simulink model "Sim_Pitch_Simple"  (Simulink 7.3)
settings: Solver=ode23s  StartTime=0.0  StopTime=1000  RelTol=1e-3
InitFcn:
  | init
StartFcn:
  | init
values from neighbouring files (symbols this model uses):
  d2r = pi/180    (= 0.0174532925199)    [init.m]    (also in robust.m)
  r2d = 180/pi    (= 57.2957795131)    [init.m]    (also in robust.m)
undefined symbols (not defined in the file or in its folder): Aps, Bps, Cps, Dps, Kmix, Kq

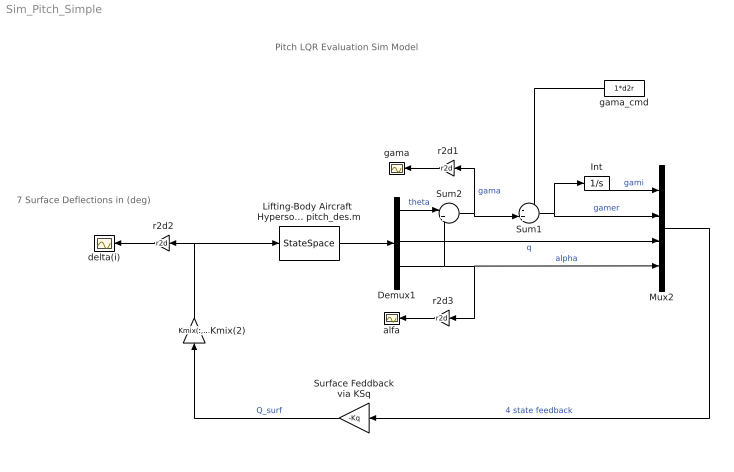
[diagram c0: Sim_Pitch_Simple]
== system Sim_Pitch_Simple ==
  note: 7 Surface Deflections in (deg)
  note: Pitch LQR Evaluation Sim Model
  " r2d1" : Gain  Gain=r2d  ParameterDataType=sfix(16)  ParameterScaling=2^0  OutDataType=sfix(16)  OutScaling=2^0
  " r2d2" : Gain  Gain=r2d  ParameterDataType=sfix(16)  ParameterScaling=2^0  OutDataType=sfix(16)  OutScaling=2^0
  " r2d3" : Gain  Gain=r2d  ParameterDataType=sfix(16)  ParameterScaling=2^0  OutDataType=sfix(16)  OutScaling=2^0
  Demux1 : Demux  Outputs=3
  Int : Integrator
  Kmix(2) : Gain  Gain=Kmix(:,2)  Multiplication=Matrix(K*u)  ParameterDataType=sfix(16)  ParameterScaling=2^0  OutDataType=sfix(16)  OutScaling=2^0
  Lifting-Body Aircraft  Hypersonic Pitch  Design Model from file pitch_des.m : StateSpace  A=Aps  B=Bps  C=Cps  D=Dps
  Mux2 : Mux
  Sum1 : Sum  Inputs=-+|  OutDataType=sfix(16)  OutScaling=2^0
  Sum2 : Sum  Inputs=|+-  OutDataType=sfix(16)  OutScaling=2^0
  Surface Feddback via KSq : Gain  Gain=-Kq  Multiplication=Matrix(K*u)  ParameterDataType=sfix(16)  ParameterScaling=2^0  OutDataType=sfix(16)  OutScaling=2^0
  alfa : Scope
  delta(i) : Scope
  gama : Scope
  gama_cmd : Constant  Value=1*d2r  OutDataType=sfix(16)  OutScaling=2^0
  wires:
  Demux1/2 -> Mux2/3  "q"
  Mux2/1 -> Surface Feddback via KSq/1  "4 state feedback"
  Surface Feddback via KSq/1 -> Kmix(2)/1  "Q_surf"
  Lifting-Body Aircraft  Hypersonic Pitch  Design Model from file pitch_des.m/1 -> Demux1/1
  Demux1/3 -> Sum2/2, Mux2/4, " r2d3"/1  "alpha"
  Demux1/1 -> Sum2/1  "theta"
  Sum2/1 -> " r2d1"/1, Sum1/2  "gama"
  " r2d1"/1 -> gama/1
  Kmix(2)/1 -> Lifting-Body Aircraft  Hypersonic Pitch  Design Model from file pitch_des.m/1, " r2d2"/1
  " r2d2"/1 -> delta(i)/1
  Int/1 -> Mux2/1  "gami"
  Sum1/1 -> Mux2/2, Int/1  "gamer"
  gama_cmd/1 -> Sum1/1
  " r2d3"/1 -> alfa/1
